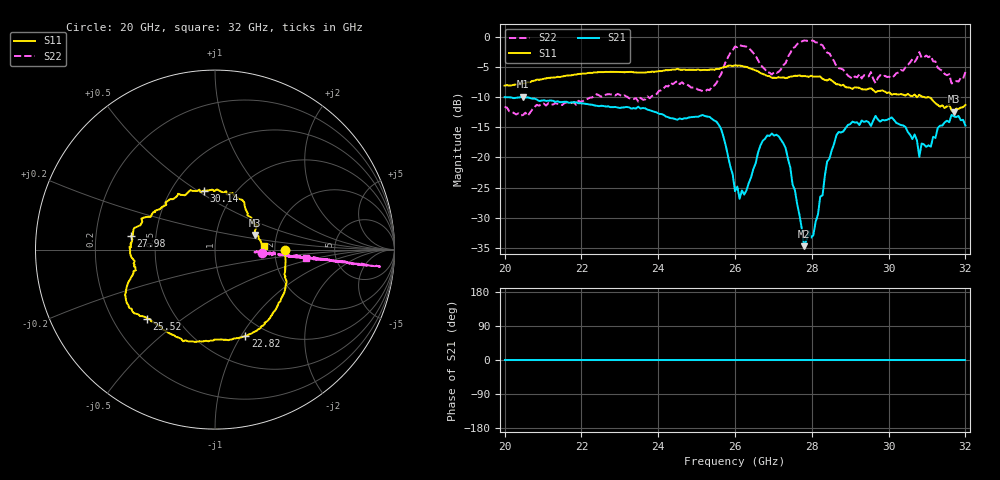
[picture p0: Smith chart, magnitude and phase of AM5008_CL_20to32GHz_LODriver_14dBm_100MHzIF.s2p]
!Keysight Technologies,N5245B,MY58422270,A.16.20.02
!Mixer S2P File: Scalar Mixer Measurement
!Calibration State: On
!Parameters: Stimulus Freq, S11, SC21, SC12, S22
# Hz  S  DB  R  50.0
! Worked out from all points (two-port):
!   201 points, 20 GHz to 32 GHz, reference 50 ohm
!   highest |S21| = -9.97 dB at 20.48 GHz (marker M1); lowest = -34.7 dB at 27.8 GHz (marker M2)
!   |S21| within 3 dB of the highest: start of sweep to 24.14 GHz; 31.6398 GHz to 31.64101 GHz (1.207 MHz wide, 0.00381 % of centre)
!   lowest |S11| = -12.4 dB at 31.7 GHz (marker M3), VSWR 1.63, Z = 77.5 + j13.4 ohm
!   |S11| at or under -10 dB: 30.73314 GHz to 30.74743 GHz (14.3 MHz wide, 0.0465 % of centre); 30.92 GHz to end of sweep
!   |S22| runs from -13.1 to -0.7 dB; largest |S21 - S12| = 0.32
!   S11 on the Smith chart (normalised r, x): 20 GHz: 2.29, +0.00; 22.82 GHz: 0.80, -1.04; 25.52 GHz: 0.35, -0.38; 27.98 GHz: 0.36, +0.07; 30.14 GHz: 0.72, +0.53; 32 GHz: 1.74, +0.08
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2e10  -8.13 0.0  -10.04 0.0  -200.00 90.0  -11.64 -4.5
2.048e10  -7.75 -17.7  -9.97 0.0  -200.00 90.0  -12.99 -4.3
2.204e10  -6.14 -54.2  -11.06 0.0  -200.00 90.0  -10.67 -4.3
2.282e10  -5.84 -70.7  -11.68 0.0  -200.00 90.0  -9.59 -3.5
2.402e10  -5.73 -98.3  -12.79 0.0  -200.00 90.0  -8.99 -4.1
2.552e10  -5.36 -134.5  -14.10 0.0  -200.00 90.0  -7.67 -5.4
2.6e10  -4.76 -145.9  -25.58 0.0  -200.00 90.0  -1.66 -6.0
2.624e10  -4.99 -152.2  -26.14 0.0  -200.00 90.0  -1.61 -6.1
2.672e10  -6.19 -162.0  -17.27 0.0  -200.00 90.0  -5.06 -4.4
2.714e10  -6.73 -168.3  -16.53 0.0  -200.00 90.0  -5.82 -4.7
2.744e10  -6.63 -174.6  -21.66 0.0  -200.00 90.0  -2.74 -5.4
2.78e10  -6.54 175.7  -34.68 0.0  -200.00 90.0  -0.65 -5.8
2.798e10  -6.48 170.8  -33.26 0.0  -200.00 90.0  -0.68 -5.8
2.804e10  -6.65 170.7  -32.85 0.0  -200.00 90.0  -0.69 -6.0
2.84e10  -7.26 159.1  -20.67 0.0  -200.00 90.0  -2.68 -5.4
2.864e10  -7.89 153.2  -16.33 0.0  -200.00 90.0  -4.91 -5.7
3.002e10  -9.24 104.7  -13.57 0.0  -200.00 90.0  -6.66 -4.9
3.014e10  -9.51 100.8  -13.79 0.0  -200.00 90.0  -6.53 -4.5
3.068e10  -9.60 79.1  -16.20 0.0  -200.00 90.0  -4.21 -4.9
3.08e10  -9.64 72.7  -19.93 0.0  -200.00 90.0  -2.56 -5.3
3.17e10  -12.44 20.0  -13.21 0.0  -200.00 90.0  -7.67 -5.2
3.2e10  -11.31 4.3  -14.73 0.0  -200.00 90.0  -5.89 -5.6
